
DATA_BLOCK DB3476
TITLE=
VERSION : 0.1

STRUCT
   CM_ID : STRING  [8 ] := '=PRM'; //COMPOSITE MACHINE
   STATION_ID : STRING  [8 ] := '++OP10'; //STATION - TRATTO - ZONE
   ELEMENT_ID : STRING  [8 ] := '+81VA41'; //ELEMENT
   DB_ID : INT := 0 ; //DB SIZE OR TYPE
   PART_STYLE : STRING  [12 ]; //PART STYLE ON LAST STATION
   ACT_CYCLE_TIME : INT ; //ACTUAL CYCLE TIME FOR THIS STYLE
   COUNT_GOOD : INT ; //COUNTER GOOD PIECES
   COUNT_SCRAP : INT ; //COUNTER SCRAP PIECES
   SPARE_00 : ARRAY  [0 .. 15 ] OF //SPARE INTEGER
   INT ;
   SPARE_01 : ARRAY  [0 .. 17 ] OF //SPARE INTEGER
   INT ;
   CODE_EVENT : ARRAY  [0 .. 7 ] OF //CODE EVENT - EXTENDED FAULT CODE DIAGNOSTIC
   INT ;
   EVENT : STRUCT
      E0000 : BOOL ; //+81VA41-M1;MS.GENERALI ERRORE;1

E0001 : BOOL ; //+81VA41-M1;MS.GENERALI AVVERTIMENTO;2

E0002 : BOOL ; //+81VA41-M1;MS.MODALITA MANUALE;16

E0003 : BOOL ; //+81VA41-M1;MS.MODO AUTOMATICO;19

E0004 : BOOL ; //+81VA41-M1;MS.RILASCIO;17

E0005 : BOOL ; //+81VA41-M1; MS. APERTO;58

E0006 : BOOL ; //+81VA41-M1; MS. VICINO;58

E0007 : BOOL ; //+81VA41-M1; MS. FUNZIONARE;58

E0008 : BOOL ; //+81VA41-M1; MS. APERTURA;58

E0009 : BOOL ; //+81VA41-M1; MS. CHIUSURA;58

E0010 : BOOL ; //+81VA41-M1; MS. ERA APERTO;58

E0011 : BOOL ; //+81VA41-M1; MS. ERA CHIUSO;58

E0012 : BOOL ; //+81VA41-M1; MS. MS_14;58

E0013 : BOOL ; //+81VA41-M1; MS. MS_15;58

E0014 : BOOL ; //+81VA41-M1; MS. MS_16;58

E0015 : BOOL ; //+81VA41-M1; MS. MS_17;58

E0016 : BOOL ; //+81VA41-M1;ME.DURATA APERTURA ERRORE;1

E0017 : BOOL ; //+81VA41-M1;ME.DURATA CHIUSURA ERRORE;1

E0018 : BOOL ; //+81VA41-M1;ME.VALIDITA;1

E0019 : BOOL ; //+81VA41-M1;ME.FUSIBILE;1

E0020 : BOOL ; //+81VA41-M1;ME.PLAUSIBILITA APERTO;1

E0021 : BOOL ; //+81VA41-M1;ME.PLAUSIBILITA CHIUDI;1

E0022 : BOOL ; //+81VA41-M1; ME. ME_06;58

E0023 : BOOL ; //+81VA41-M1; ME. ME_07;58

E0024 : BOOL ; //+81VA41-M1; ME. ME_10;58

E0025 : BOOL ; //+81VA41-M1; ME. ME_11;58

E0026 : BOOL ; //+81VA41-M1; ME. ME_12;58

E0027 : BOOL ; //+81VA41-M1; ME. ME_13;58

E0028 : BOOL ; //+81VA41-M1; ME. ME_14;58

E0029 : BOOL ; //+81VA41-M1; ME. ME_15;58

E0030 : BOOL ; //+81VA41-M1; ME. ME_16;58

E0031 : BOOL ; //+81VA41-M1; ME. ME_17;58
E0032 : BOOL ; //+81VA41-M2;MS.GENERALI ERRORE;1
E0033 : BOOL ; //+81VA41-M2;MS.GENERALI AVVERTIMENTO;2
E0034 : BOOL ; //+81VA41-M2;MS.MODALITA MANUALE;16
E0035 : BOOL ; //+81VA41-M2;MS.MODO AUTOMATICO;19
E0036 : BOOL ; //+81VA41-M2;MS.RILASCIO;17
E0037 : BOOL ; //+81VA41-M2; MS. APERTO;58
E0038 : BOOL ; //+81VA41-M2; MS. VICINO;58
E0039 : BOOL ; //+81VA41-M2; MS. FUNZIONARE;58
E0040 : BOOL ; //+81VA41-M2; MS. APERTURA;58
E0041 : BOOL ; //+81VA41-M2; MS. CHIUSURA;58
E0042 : BOOL ; //+81VA41-M2; MS. ERA APERTO;58
E0043 : BOOL ; //+81VA41-M2; MS. ERA CHIUSO;58
E0044 : BOOL ; //+81VA41-M2; MS. MS_14;58
E0045 : BOOL ; //+81VA41-M2; MS. MS_15;58
E0046 : BOOL ; //+81VA41-M2; MS. MS_16;58
E0047 : BOOL ; //+81VA41-M2; MS. MS_17;58
E0048 : BOOL ; //+81VA41-M2;ME.DURATA APERTURA ERRORE;1
E0049 : BOOL ; //+81VA41-M2;ME.DURATA CHIUSURA ERRORE;1
E0050 : BOOL ; //+81VA41-M2;ME.VALIDITA;1
E0051 : BOOL ; //+81VA41-M2;ME.FUSIBILE;1
E0052 : BOOL ; //+81VA41-M2;ME.PLAUSIBILITA APERTO;1
E0053 : BOOL ; //+81VA41-M2;ME.PLAUSIBILITA CHIUDI;1
E0054 : BOOL ; //+81VA41-M2; ME. ME_06;58
E0055 : BOOL ; //+81VA41-M2; ME. ME_07;58
E0056 : BOOL ; //+81VA41-M2; ME. ME_10;58
E0057 : BOOL ; //+81VA41-M2; ME. ME_11;58
E0058 : BOOL ; //+81VA41-M2; ME. ME_12;58
E0059 : BOOL ; //+81VA41-M2; ME. ME_13;58
E0060 : BOOL ; //+81VA41-M2; ME. ME_14;58
E0061 : BOOL ; //+81VA41-M2; ME. ME_15;58
E0062 : BOOL ; //+81VA41-M2; ME. ME_16;58
E0063 : BOOL ; //+81VA41-M2; ME. ME_17;58
END_STRUCT;
END_STRUCT;
BEGIN
CM_ID := '=PRM';
STATION_ID := '++OP10';
ELEMENT_ID := '+81VA41';
DB_ID := 0 ;
PART_STYLE := '';
ACT_CYCLE_TIME := 0;
COUNT_GOOD := 0;
COUNT_SCRAP := 0;
SPARE_00[0] := 0;
SPARE_00[1] := 0;
SPARE_00[2] := 0;
SPARE_00[3] := 0;
SPARE_00[4] := 0;
SPARE_00[5] := 0;
SPARE_00[6] := 0;
SPARE_00[7] := 0;
SPARE_00[8] := 0;
SPARE_00[9] := 0;
SPARE_00[10] := 0;
SPARE_00[11] := 0;
SPARE_00[12] := 0;
SPARE_00[13] := 0;
SPARE_00[14] := 0;
SPARE_00[15] := 0;
SPARE_01[0] := 0;
SPARE_01[1] := 0;
SPARE_01[2] := 0;
SPARE_01[3] := 0;
SPARE_01[4] := 0;
SPARE_01[5] := 0;
SPARE_01[6] := 0;
SPARE_01[7] := 0;
SPARE_01[8] := 0;
SPARE_01[9] := 0;
SPARE_01[10] := 0;
SPARE_01[11] := 0;
SPARE_01[12] := 0;
SPARE_01[13] := 0;
SPARE_01[14] := 0;
SPARE_01[15] := 0;
SPARE_01[16] := 0;
SPARE_01[17] := 0;
CODE_EVENT[0] := 0;
CODE_EVENT[1] := 0;
CODE_EVENT[2] := 0;
CODE_EVENT[3] := 0;
CODE_EVENT[4] := 0;
CODE_EVENT[5] := 0;
CODE_EVENT[6] := 0;
CODE_EVENT[7] := 0;
EVENT.E0000 := FALSE;
EVENT.E0001 := FALSE;
EVENT.E0002 := FALSE;
EVENT.E0003 := FALSE;
EVENT.E0004 := FALSE;
EVENT.E0005 := FALSE;
EVENT.E0006 := FALSE;
EVENT.E0007 := FALSE;
EVENT.E0008 := FALSE;
EVENT.E0009 := FALSE;
EVENT.E0010 := FALSE;
EVENT.E0011 := FALSE;
EVENT.E0012 := FALSE;
EVENT.E0013 := FALSE;
EVENT.E0014 := FALSE;
EVENT.E0015 := FALSE;
EVENT.E0016 := FALSE;
EVENT.E0017 := FALSE;
EVENT.E0018 := FALSE;
EVENT.E0019 := FALSE;
EVENT.E0020 := FALSE;
EVENT.E0021 := FALSE;
EVENT.E0022 := FALSE;
EVENT.E0023 := FALSE;
EVENT.E0024 := FALSE;
EVENT.E0025 := FALSE;
EVENT.E0026 := FALSE;
EVENT.E0027 := FALSE;
EVENT.E0028 := FALSE;
EVENT.E0029 := FALSE;
EVENT.E0030 := FALSE;
EVENT.E0031 := FALSE;
EVENT.E0032 := FALSE;
EVENT.E0033 := FALSE;
EVENT.E0034 := FALSE;
EVENT.E0035 := FALSE;
EVENT.E0036 := FALSE;
EVENT.E0037 := FALSE;
EVENT.E0038 := FALSE;
EVENT.E0039 := FALSE;
EVENT.E0040 := FALSE;
EVENT.E0041 := FALSE;
EVENT.E0042 := FALSE;
EVENT.E0043 := FALSE;
EVENT.E0044 := FALSE;
EVENT.E0045 := FALSE;
EVENT.E0046 := FALSE;
EVENT.E0047 := FALSE;
EVENT.E0048 := FALSE;
EVENT.E0049 := FALSE;
EVENT.E0050 := FALSE;
EVENT.E0051 := FALSE;
EVENT.E0052 := FALSE;
EVENT.E0053 := FALSE;
EVENT.E0054 := FALSE;
EVENT.E0055 := FALSE;
EVENT.E0056 := FALSE;
EVENT.E0057 := FALSE;
EVENT.E0058 := FALSE;
EVENT.E0059 := FALSE;
EVENT.E0060 := FALSE;
EVENT.E0061 := FALSE;
EVENT.E0062 := FALSE;
EVENT.E0063 := FALSE;
END_DATA_BLOCK
